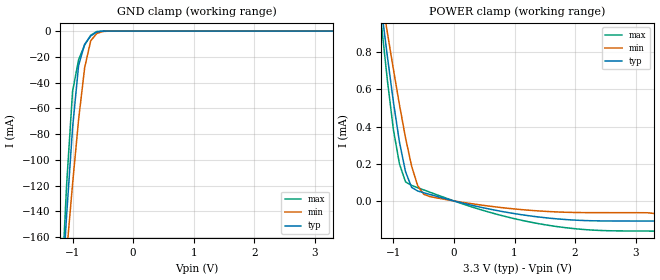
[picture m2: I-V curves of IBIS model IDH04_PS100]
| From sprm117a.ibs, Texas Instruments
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[Model]   IDH04_PS100
Model_type   Input
Polarity   Non-Inverting
| signals   A, Y
Vinl = 0.8V
Vinh = 2.0V
|   typ   min   max
C_comp   1.6130p   1.5354p   1.7989p
|   typ   min   max
[Temperature Range]   25   -40   125
|   typ   min   max
[Voltage Range]   3.30V   3.00V   3.60V
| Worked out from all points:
|   GND clamp passes 1 mA (typ) near -0.61 V on its own axis
|   POWER clamp passes 1 mA (typ) near -1.19 V on its own axis
[GND_clamp]
|   Voltage   I(typ)   I(min)   I(max)
-3.3V     -2.006A    -1.517A    -2.602A
-1.2V     -221.2mA   -230.2mA   -219.3mA
-1.1V     -144.6mA   -173.4mA   -120.9mA
-1V       -75.24mA   -118.9mA   -46.85mA
-900mV    -26.57mA   -68.74mA   -22.24mA
-800mV    -10.22mA   -28.36mA   -10.81mA
-700mV    -3.768mA   -7.528mA   -3.182mA
-600mV    -734.7uA   -1.835mA   -363.9uA
-500mV    -67.23uA   -328.9uA   -17.02uA
-400mV    -3.755uA   -40.45uA   -379.8nA
3.3V      222pA      34.33nA    0A
[POWER_clamp]
|   Voltage   I(typ)   I(min)   I(max)
-3.3V     6.84mA     5.575mA    7.993mA
-1.2V     1.035mA    1.107mA    954uA
-1.1V     777uA      904.8uA    648.8uA
-1V       531.2uA    707.1uA    381.7uA
-900mV    315.2uA    516.3uA    198.5uA
-800mV    157.1uA    338.6uA    102.3uA
-700mV    72.87uA    187.6uA    83.49uA
-600mV    53.6uA     82.48uA    71.35uA
-500mV    44.08uA    35.96uA    59.29uA
500mV     -38.01uA   -24.41uA   -52.73uA
1.4V      -86.37uA   -53.79uA   -122.3uA
3.3V      -108.3uA   -67.2uA    -162.1uA
